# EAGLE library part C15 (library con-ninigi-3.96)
NINIGI
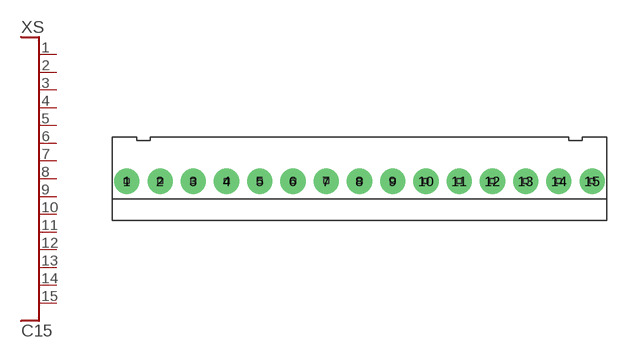
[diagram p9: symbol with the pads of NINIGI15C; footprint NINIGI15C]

Designator prefix XS

## C15  [NINIGI15C]
1  P$1
2  P$2
3  P$3
4  P$4
5  P$5
6  P$6
7  P$7
8  P$8
9  P$9
10  P$10
11  P$11
12  P$12
13  P$13
14  P$14
15  P$15

## Footprint NINIGI15C (pad centres in mm)
drill 1.6 pad 3: 1 -27.72,0; 2 -23.76,0; 3 -19.8,0; 4 -15.84,0; 5 -11.88,0; 6 -7.92,0; 7 -3.96,0; 8 0,0; 9 3.96,0; 10 7.92,0; 11 11.88,0; 12 15.84,0; 13 19.8,0; 14 23.76,0; 15 27.72,0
